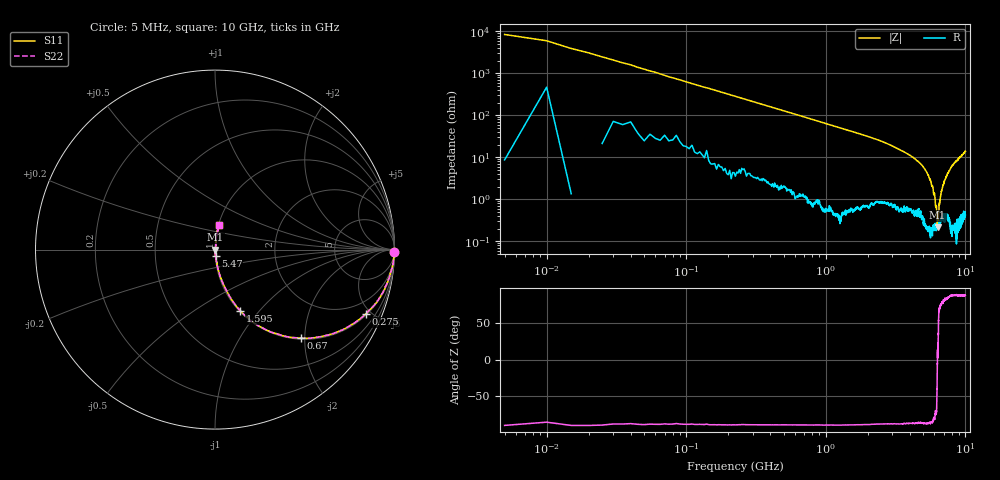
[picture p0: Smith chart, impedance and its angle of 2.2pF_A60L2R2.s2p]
! Amotech Co.,Ltd.
! http://www.amotech.co.kr/
! Part Number: A60L2R2
! These Parameters are Measured in Series Mode Connection
! Operation Temp=25[degC], DC Bias Voltage=0[V]
! Freq. Start=5[MHz] Stop=10[GHz], 2000[Steps]
! Date: Monday, July 14, 2020, 09:29:09
# GHZ S RI R 50.000000
!Freq.(Hz) S11(Real) S11(Imag) S21(Real) S21(Imag) S12(Real) S12(Imag) S22(Real) S22(Imag)
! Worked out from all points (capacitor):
!   2000 points, 5 MHz to 10 GHz, reference 50 ohm
!   read as one part in series: C = 2.53 pF near 55 MHz
!   lowest |Z| = 217 mohm at 6.32 GHz (marker M1)
!   series resonance near 6.307 GHz, so ESL is about 250 pH
!   S11 on the Smith chart (normalised r, x): 5 MHz: open; 275 MHz: 1.08, -4.65; 670 MHz: 1.02, -1.92; 1.595 GHz: 1.01, -0.80; 5.47 GHz: 1.00, -0.07; 10 GHz: 1.01, +0.28
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0.005  0.9998 -0.0118  0.000151 0.0118  0.000151 0.0118  0.9998 -0.0118
0.065  0.9871 -0.1006  0.0129 0.1006  0.0129 0.1006  0.9871 -0.1006
0.1  0.9712 -0.1535  0.0288 0.1535  0.0288 0.1535  0.9712 -0.1535
0.17  0.9309 -0.2449  0.0691 0.2449  0.0691 0.2449  0.9309 -0.2449
0.275  0.8398 -0.3581  0.1602 0.3581  0.1602 0.3581  0.8398 -0.3581
0.67  0.4799 -0.4933  0.5201 0.4933  0.5201 0.4933  0.4799 -0.4933
1.06  0.2688 -0.4375  0.7312 0.4375  0.7312 0.4375  0.2688 -0.4375
1.595  0.1411 -0.3411  0.8589 0.3411  0.8589 0.3411  0.1411 -0.3411
1.675  0.1301 -0.328  0.8699 0.328  0.8699 0.328  0.1301 -0.328
3.34  0.0285 -0.1499  0.9715 0.1499  0.9715 0.1499  0.0285 -0.1499
5.005  0.006 -0.0577  0.994 0.0577  0.994 0.0577  0.006 -0.0577
5.47  0.003 -0.0344  0.997 0.0344  0.997 0.0344  0.003 -0.0344
6.02  0.00211 -0.0134  0.9979 0.0134  0.9979 0.0134  0.00211 -0.0134
6.11  0.00246 -0.00691  0.9975 0.00691  0.9975 0.00691  0.00246 -0.00691
6.195  0.00217 -0.0067  0.9978 0.0067  0.9978 0.0067  0.00217 -0.0067
6.32  0.00214 0.000366  0.9979 -0.000366  0.9979 -0.000366  0.00214 0.000366
6.385  0.00219 0.000852  0.9978 -0.000852  0.9978 -0.000852  0.00219 0.000852
6.505  0.00297 0.00708  0.997 -0.00708  0.997 -0.00708  0.00297 0.00708
6.67  0.00351 0.0125  0.9965 -0.0125  0.9965 -0.0125  0.00351 0.0125
7.275  0.00493 0.0343  0.9951 -0.0343  0.9951 -0.0343  0.00493 0.0343
8.335  0.00744 0.0719  0.9926 -0.0719  0.9926 -0.0719  0.00744 0.0719
10  0.0232 0.1361  0.9768 -0.1361  0.9768 -0.1361  0.0232 0.1361
